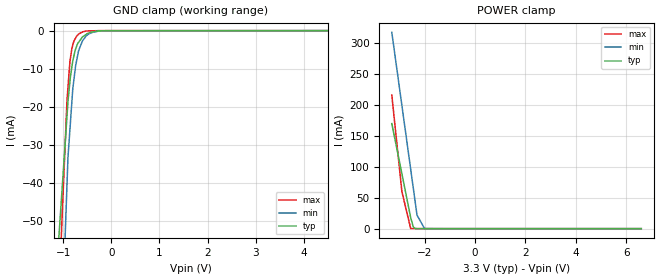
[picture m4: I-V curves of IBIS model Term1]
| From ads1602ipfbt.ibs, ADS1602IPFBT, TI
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[Model] Term1
Model_type Terminator
C_comp 2.00000pF 2.00000pF 2.00000pF
| variable typ   min   max
[Voltage Range] 3.30000V 3.00000V 3.60000V
[POWER Clamp Reference] 3.30000V 3.00000V 3.60000V
[GND Clamp Reference] 0.00000V 0.00000V 0.00000V
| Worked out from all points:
|   GND clamp passes 1 mA (typ) near -0.52 V on its own axis
|   POWER clamp passes 1 mA (typ) near -2.41 V on its own axis
[GND Clamp]
-3.3V     -470.8mA   -882.9mA   -737mA
-920mV    -22.44mA   -40.4mA    -18.29mA
-900mV    -18.67mA   -33.32mA   -14.93mA
-860mV    -13.46mA   -26.11mA   -8.212mA
-820mV    -9.641mA   -18.9mA    -4.769mA
-800mV    -7.962mA   -15.29mA   -3.814mA
-740mV    -4.792mA   -9.123mA   -1.903mA
-680mV    -3.072mA   -5.296mA   -918uA
-620mV    -2.016mA   -3.366mA   -479.1uA
-460mV    -580uA     -810.9uA   -70.72uA
-130mV    -13.65uA   -25.11uA   -1.724uA
6.6V      3.8uA      18.07uA    3.849uA
[POWER Clamp]
-3.3V     169.4mA    316.4mA    215.3mA
-2.9V     88.39mA    198.6mA    59.79mA
-2.55V    17.48mA    95.52mA    74.46uA
-2.45V    3.226mA    66.06mA    69.14uA
-2.4V     722.1uA    51.33mA    66.48uA
-2.3V     37.3uA     21.88mA    61.17uA
-2V       27.57uA    52.51uA    45.21uA
6.6V      0A         0A         0A
